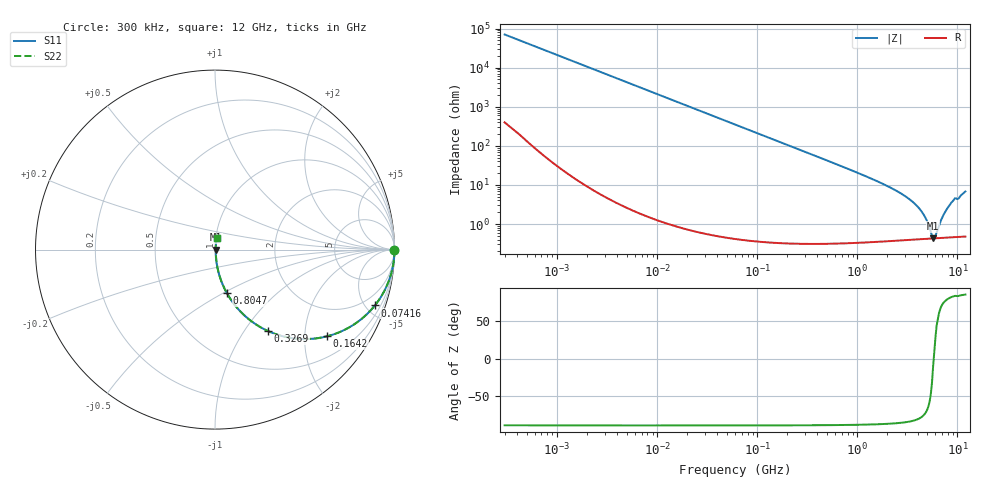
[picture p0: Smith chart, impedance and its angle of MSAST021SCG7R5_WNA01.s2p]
! MSAST021SCG7R5_WNA01  S-PARAMETER MODEL  ( General Type )
! Model Generated by TAIYO YUDEN Corporation (http://www.ty-top.com)
! Version 2.0
! TAIYO YUDEN Control No. 181101
! Copyright(c) 2015 TAIYO YUDEN CO.,LTD. All Rights Reserved.
! Product Description (link to TY-COMPAS)
! https://ds.yuden.co.jp/TYCOMPAS/or/detail?pn=MSAST021SCG7R5CWNA01&u=M
! Products Name : Multilayer Ceramic Capacitors
! Characteristics :
!  Capacitance : 7.5 pF , Rated Voltage : 25V , TCC : CG / C0G
!  Case Size : 0.25 x 0.125 / 0.0098 x 0.0049 [mm/inch] , Thickness : 0.125 / 0.0049 [mm/inch]
!  (Conditions: Temperature = 25 degC , DC Bias Current/Voltage = 0A / 0V)
! External Node Assignments :
!  1  o---| |---o  2
! GND o---------o GND
! Frequency Range : 0.3MHz  -  12000MHz  [ 401 STEP ]
# MHz S RI R 50
! Freq[MHz].  S11 Real  S11 Imag  S21 Real  S21 Imag  S12 Real  S12 Imag  S22 Real  S22 Imag
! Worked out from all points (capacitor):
!   401 points, 300 kHz to 12 GHz, reference 50 ohm
!   read as one part in series: C = 7.5 pF near 316.3 kHz
!   lowest |Z| = 435 mohm at 5.715 GHz (marker M1)
!   series resonance near 5.795 GHz, so ESL is about 100 pH
!   S11 on the Smith chart (normalised r, x): 300 kHz: open; 74.16 MHz: 1.01, -5.72; 164.2 MHz: 1.01, -2.58; 326.9 MHz: 1.01, -1.29; 804.7 MHz: 1.01, -0.52; 12 GHz: 1.01, +0.14
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0.3  1 -0.00141  9.97e-06 0.00141  9.97e-06 0.00141  1 -0.00141
1.769972  0.9999 -0.00834  7.73e-05 0.00834  7.73e-05 0.00834  0.9999 -0.00834
10.44266  0.9976 -0.0491  0.00244 0.0491  0.00244 0.0491  0.9976 -0.0491
27.10171  0.9839 -0.1256  0.0161 0.1256  0.0161 0.1256  0.9839 -0.1256
60  0.9257 -0.2617  0.0743 0.2617  0.0743 0.2617  0.9257 -0.2617
74.16388  0.8908 -0.3112  0.1092 0.3112  0.1092 0.3112  0.8908 -0.3112
110.3493  0.7866 -0.4088  0.2134 0.4088  0.2134 0.4088  0.7866 -0.4088
164.1901  0.6248 -0.4829  0.3752 0.4829  0.3752 0.4829  0.6248 -0.4829
326.9496  0.296 -0.4541  0.704 0.4541  0.704 0.4541  0.296 -0.4541
353.9943  0.264 -0.4382  0.736 0.4382  0.736 0.4382  0.264 -0.4382
526.7124  0.1396 -0.3427  0.8604 0.3427  0.8604 0.3427  0.1396 -0.3427
804.7407  0.0653 -0.2409  0.9347 0.2409  0.9347 0.2409  0.0653 -0.2409
2088.533  0.0113 -0.087  0.9887 0.087  0.9887 0.087  0.0113 -0.087
3107.553  0.00619 -0.048  0.9938 0.048  0.9938 0.048  0.00619 -0.048
4050.141  0.00474 -0.0264  0.9953 0.0264  0.9953 0.0264  0.00474 -0.0264
4747.894  0.00435 -0.0144  0.9956 0.0144  0.9956 0.0144  0.00435 -0.0144
5715.274  0.00427 -0.000763  0.9957 0.000763  0.9957 0.000763  0.00427 -0.000763
6026.253  0.00431 0.00227  0.9957 -0.00227  0.9957 -0.00227  0.00431 0.00227
7064.448  0.00461 0.0141  0.9954 -0.0141  0.9954 -0.0141  0.00461 0.0141
8281.503  0.00535 0.0289  0.9946 -0.0289  0.9946 -0.0289  0.00535 0.0289
9207.246  0.0063 0.0412  0.9937 -0.0412  0.9937 -0.0412  0.0063 0.0412
12000  0.00929 0.067  0.9907 -0.067  0.9907 -0.067  0.00929 0.067
